(* Logix 5000 AddOnInstructionDefinition export B256_NRED; software revision 30.00 *)

ADD_ON_INSTRUCTION D_SHR   (* revision 1.0, vendor Ken Fischer, NSWCPD, C512 *)
// DINT bit shift right of the 32-bit argument Inp_A by Inp_B bits with paddding by zeros on the right
// Revision note:
// Rev1.0: TBD - Initial Release
VAR_IN_OUT
   Inp_A : DINT; {required}   // 64-bit Integer to be right circular rotated
END_VAR
VAR_INPUT
   Inp_B : INT; {required}   // Number of bits to shift
END_VAR
VAR_IN_OUT
   Out : DINT; {required}   // Result
END_VAR
VAR
   BSR_Cntrl : CONTROL := (LEN := 32);
   ONS : BOOL;
   Source_Bit : BOOL;
   Wrk_InpA : DINT[2];
END_VAR

ROUTINE Logic   (* ladder *)
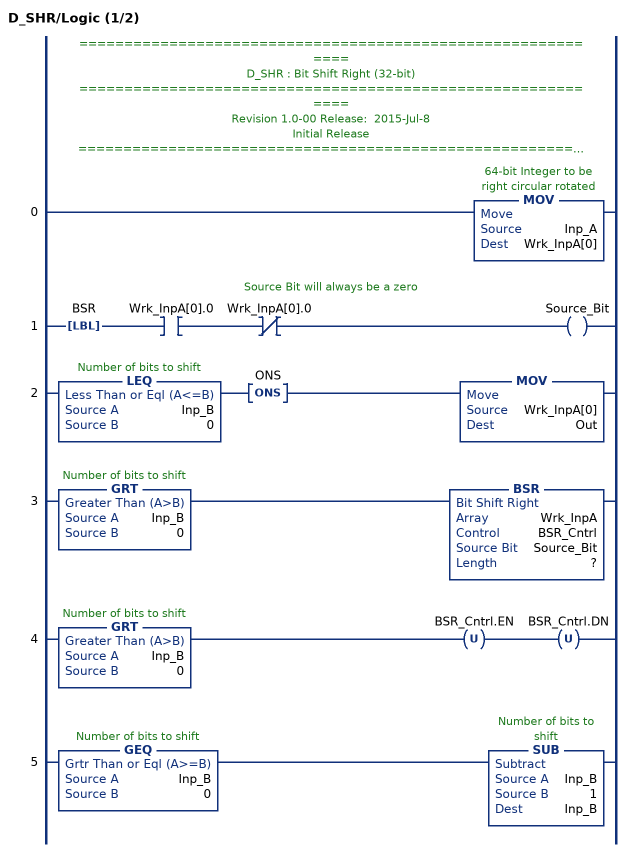
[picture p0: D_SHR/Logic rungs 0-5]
   // ============================================================
   // D_SHR : Bit Shift Right (32-bit)
   // ============================================================
   // Revision 1.0-00 Release:  2015-Jul-8
   // Initial Release
   // ============================================================
   // Performs a right bit shift of the 32-bit argument Inp_A by the
   // number of bits defined in the 16-bit argument Inp_B, with padding by zeros.
   0: MOV(Inp_A,Wrk_InpA[0]);
   // Source Bit will always be a zero
   1: LBL(BSR)XIC(Wrk_InpA[0].0)XIO(Wrk_InpA[0].0)OTE(Source_Bit);
   2: LEQ(Inp_B,0)ONS(ONS)MOV(Wrk_InpA[0],Out);
   3: GRT(Inp_B,0)BSR(Wrk_InpA,BSR_Cntrl,Source_Bit,?);
   4: GRT(Inp_B,0)OTU(BSR_Cntrl.EN)OTU(BSR_Cntrl.DN);
   5: GEQ(Inp_B,0)SUB(Inp_B,1,Inp_B);
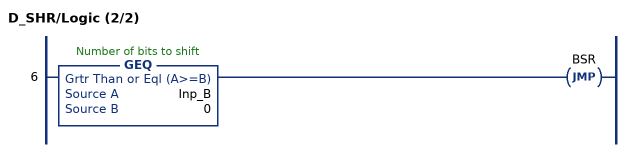
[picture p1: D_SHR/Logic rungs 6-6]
   6: GEQ(Inp_B,0)JMP(BSR);
END_ROUTINE
END_ADD_ON_INSTRUCTION

ADD_ON_INSTRUCTION B256_NRED   (* revision 1.0 20170916, vendor Kenneth A. Fischer *)
// Reduce 256-bit integer stored in 22 pieces by propagating carries
// Revision note:
// Rev1.0: 20170916 - Initial Release
VAR_IN_OUT
   Inp_C : DINT[22]; {required}
END_VAR
VAR
   D_SHR : D_SHR;
   temp : DINT;
   i : INT;
END_VAR

ROUTINE Logic   (* ladder *)
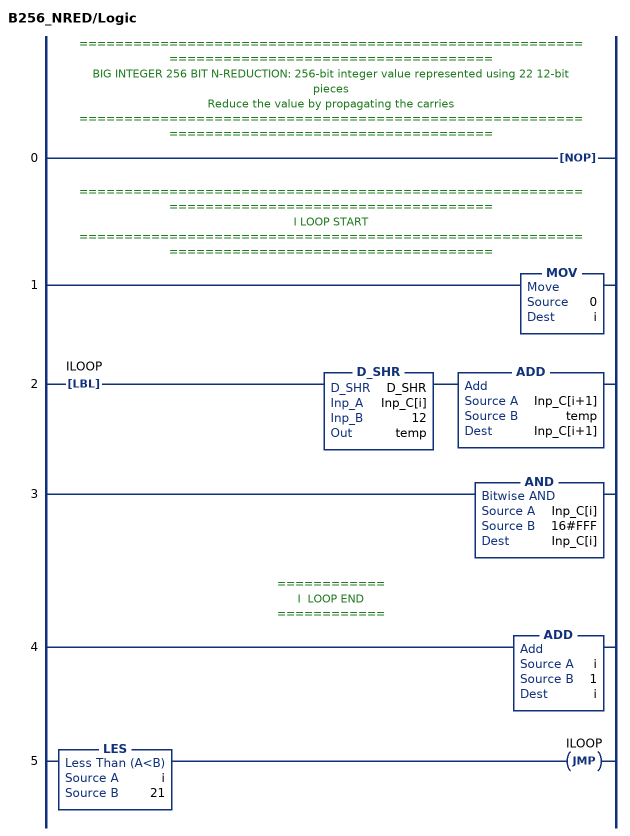
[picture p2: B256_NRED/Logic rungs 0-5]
   // ============================================================================================
   // BIG INTEGER 256 BIT N-REDUCTION: 256-bit integer value represented using 22 12-bit pieces
   // Reduce the value by propagating the carries
   // ============================================================================================
   0: NOP();
   // ============================================================================================
   // I LOOP START
   // ============================================================================================
   1: MOV(0,i);
   2: LBL(ILOOP)D_SHR(D_SHR,Inp_C[i],12,temp)ADD(Inp_C[i+1],temp,Inp_C[i+1]);
   3: AND(Inp_C[i],16#FFF,Inp_C[i]);
   // ============
   // I  LOOP END
   // ============
   4: ADD(i,1,i);
   5: LES(i,21)JMP(ILOOP);
END_ROUTINE
END_ADD_ON_INSTRUCTION
